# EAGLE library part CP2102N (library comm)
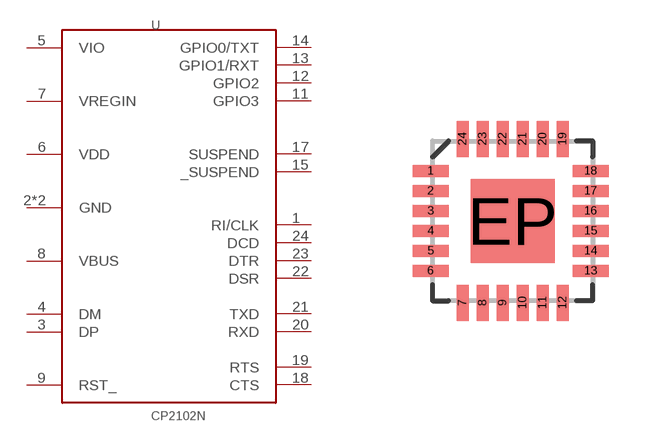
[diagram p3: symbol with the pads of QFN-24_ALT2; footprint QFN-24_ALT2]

Designator prefix U

## CP2102N  [QFN-24_ALT2]
1  RI/CLK
2  GND
3  DP
4  DM
5  VIO
6  VDD
7  VREGIN
8  VBUS
9  RST_
11  GPIO3
12  GPIO2
13  GPIO1/RXT
14  GPIO0/TXT
15  _SUSPEND
17  SUSPEND
18  CTS
19  RTS
20  RXD
21  TXD
22  DSR
23  DTR
24  DCD
EP  GND

## Footprint QFN-24_ALT2 (pad centres in mm)
24-pin QFN with Exposed Thermal pad Parts that use this package: A6282 Last modified: 8/20/10 ***UNPROVEN***
smd 0.9 x 0.3: 1 -2.05,1.25; 2 -2.05,0.75; 3 -2.05,0.25; 4 -2.05,-0.25; 5 -2.05,-0.75; 6 -2.05,-1.25; 13 1.95,-1.25; 14 1.95,-0.75; 15 1.95,-0.25; 16 1.95,0.25; 17 1.95,0.75; 18 1.95,1.25
smd 0.3 x 0.9: 7 -1.25,-2.05; 8 -0.75,-2.05; 9 -0.25,-2.05; 10 0.25,-2.05; 11 0.75,-2.05; 12 1.25,-2.05; 19 1.25,2.05; 20 0.75,2.05; 21 0.25,2.05; 22 -0.25,2.05; 23 -0.75,2.05; 24 -1.25,2.05
smd 2.1 x 2.1: EP 0,0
